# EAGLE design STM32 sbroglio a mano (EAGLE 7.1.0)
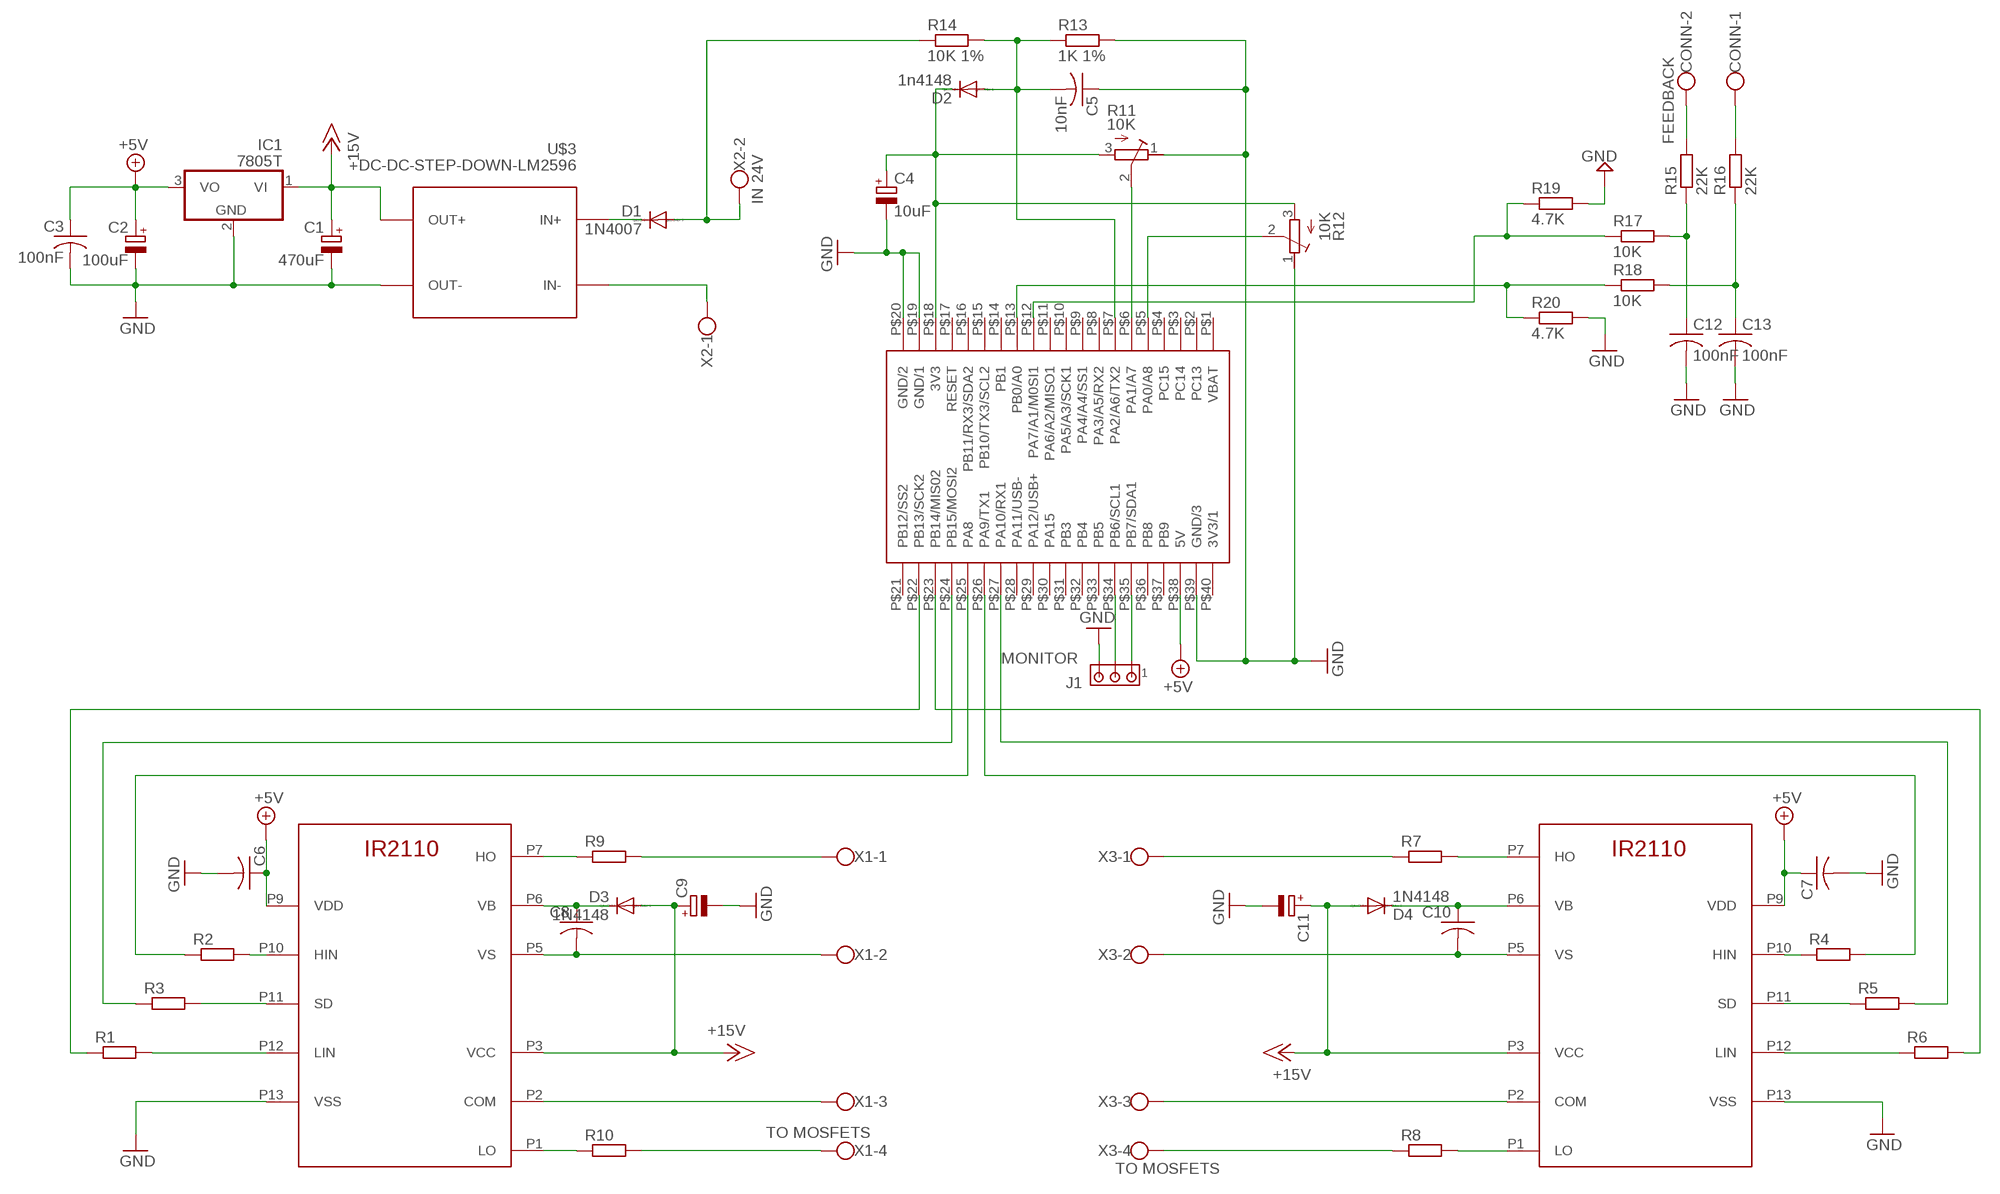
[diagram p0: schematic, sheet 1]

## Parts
C1  470uF  CPOL-EUE5-10.5  [E5-10,5]
C2  100uF  CPOL-EUE5-10.5  [E5-10,5]
C3  100nF  C-US050-025X075  [C050-025X075]
C4  10uF  CPOL-EUE3.5-8  [E3,5-8]
C5  10nF  C-US050-025X075  [C050-025X075]
C6  C-US050-025X075  [C050-025X075]
C7  C-US050-025X075  [C050-025X075]
C8  C-US050-025X075  [C050-025X075]
C9  CPOL-EUE3.5-8  [E3,5-8]
C10  C-US050-025X075  [C050-025X075]
C11  CPOL-EUE3.5-8  [E3,5-8]
C12  100nF  C-US050-025X075  [C050-025X075]
C13  100nF  C-US050-025X075  [C050-025X075]
CONN  FEEDBACK  W237-102  [W237-102]
D1  1N4007  1N4004  [DO41-10]
D2  1n4148  1N4004  [DO41-10]
D3  1N4148  1N4004  [DO41-10]
D4  1N4148  1N4004  [DO41-10]
IC1  7805T  [TO220H]
J1  MONITOR  MTA03-100  [10X03MTA]
R1  R-EU_0204/5  [0204/5]
R2  R-EU_0204/5  [0204/5]
R3  R-EU_0204/5  [0204/5]
R4  R-EU_0204/5  [0204/5]
R5  R-EU_0204/5  [0204/5]
R6  R-EU_0204/5  [0204/5]
R7  R-EU_0204/5  [0204/5]
R8  R-EU_0204/5  [0204/5]
R9  R-EU_0204/5  [0204/5]
R10  R-EU_0204/5  [0204/5]
R11  10K  R-TRIMMT93YB  [RTRIMT93YB]
R12  10K  R-TRIMMT93YA  [RTRIMT93YA]
R13  1K 1%  R-EU_0204/5  [0204/5]
R14  10K 1%  R-EU_0204/5  [0204/5]
R15  22K  R-EU_0204/5  [0204/5]
R16  22K  R-EU_0204/5  [0204/5]
R17  10K  R-EU_0204/5  [0204/5]
R18  10K  R-EU_0204/5  [0204/5]
R19  4.7K  R-EU_0204/5  [0204/5]
R20  4.7K  R-EU_0204/5  [0204/5]
U$1  IR2110N  [DIL14-1]
U$2  IR2110N  [DIL14-1]
U$3  DC-DC-STEP-DOWN-LM2596  [DC-DC-STEP-DOWN-LM2596]
U$4  BLUEPILL  [40-DIP-BLUE-PIL]
X1  TO MOSFETS  W237-4  [W237-4]
X2  IN 24V  W237-102  [W237-102]
X3  TO MOSFETS  W237-4  [W237-4]

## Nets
+5V: C2.+ C3.1 C6.1 C7.1 IC1.3(VO) U$1.P9(VDD) U$2.P9(VDD) U$4.P$38(5V)
+15V: C1.+ C9.+ C11.+ D3.A D4.A IC1.1(VI) U$1.P3(VCC) U$2.P3(VCC) U$3.OUT+
GND: C1.- C2.- C3.2 C4.- C5.1 C6.2 C7.2 C9.- C11.- C12.2 C13.2 IC1.2(GND) J1.3 R11.1(E) R12.1(E) R13.2 R19.2 R20.2 U$1.P13(VSS) U$2.P13(VSS) U$3.OUT- U$4.P$19(GND/1) U$4.P$20(GND/2) U$4.P$39(GND/3)
N$1: R2.2 U$1.P10(HIN)
N$2: R3.2 U$1.P11(SD)
N$3: R1.2 U$1.P12(LIN)
N$4: R4.1 U$2.P10(HIN)
N$5: R5.1 U$2.P11(SD)
N$6: R6.1 U$2.P12(LIN)
N$7: R2.1 U$4.P$25(PA8)
N$8: R1.1 U$4.P$22(PB13/SCK2)
N$9: R3.1 U$4.P$24(PB15/MOSI2)
N$10: R4.2 U$4.P$26(PA9/TX1)
N$11: R6.2 U$4.P$23(PB14/MIS02)
N$12: R5.2 U$4.P$27(PA10/RX1)
N$13: D1.A R14.1 X2.2
N$14: R9.1 U$1.P7(HO)
N$15: R10.1 U$1.P1(LO)
N$16: R8.2 U$2.P1(LO)
N$17: R7.2 U$2.P7(HO)
N$18: R12.2(S) U$4.P$5(PA0/A8)
N$19: R11.2(S) U$4.P$6(PA1/A7)
N$20: D1.C U$3.IN+
N$21: U$3.IN- X2.1
N$22: C4.+ D2.C R11.3(A) R12.3(A) U$4.P$18(3V3)
N$23: C5.2 D2.A R13.1 R14.2 U$4.P$7(PA2/A6/TX2)
N$24: C8.1 D3.C U$1.P6(VB)
N$25: C8.2 U$1.P5(VS) X1.2
N$26: R9.2 X1.1
N$27: U$1.P2(COM) X1.3
N$28: R10.2 X1.4
N$29: C10.1 D4.C U$2.P6(VB)
N$30: C10.2 U$2.P5(VS) X3.2
N$31: R7.1 X3.1
N$33: R8.1 X3.4
N$34: C12.1 R15.1 R17.2
N$35: C13.1 R16.1 R18.2
N$36: R18.1 R20.1 U$4.P$13(PB0/A0)
N$37: R17.1 R19.1 U$4.P$12(PA7/A1/M0SI1)
N$38: J1.2 U$4.P$34(PB6/SCL1)
N$39: J1.1 U$4.P$35(PB7/SDA1)
N$40: U$2.P2(COM) X3.3
N$42: CONN.2 R15.2
N$43: CONN.1 R16.2
Unconnected: U$4.P$1(VBAT) U$4.P$2(PC13) U$4.P$3(PC14) U$4.P$4(PC15) U$4.P$8(PA3/A5/RX2) U$4.P$9(PA4/A4/SS1) U$4.P$10(PA5/A3/SCK1) U$4.P$11(PA6/A2/MISO1) U$4.P$14(PB1) U$4.P$15(PB10/TX3/SCL2) U$4.P$16(PB11/RX3/SDA2) U$4.P$17(RESET) U$4.P$21(PB12/SS2) U$4.P$28(PA11/USB-) U$4.P$29(PA12/USB+) U$4.P$30(PA15) U$4.P$31(PB3) U$4.P$32(PB4) U$4.P$33(PB5) U$4.P$36(PB8) U$4.P$37(PB9) U$4.P$40(3V3/1)

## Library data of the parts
C1 = rcl:CPOL-EU: POLARIZED CAPACITOR, European symbol
C2 C4 C9 C11 = resistor modified:CPOL-EU: POLARIZED CAPACITOR, European symbol
C3 C5-C8 C10 C12 C13 = resistor modified:C-US: CAPACITOR, American symbol
CONN X2 = con-wago-500 modified:W237-102: WAGO SCREW CLAMP; MPN: 237-102; OC_FARNELL: unknown; OC_NEWARK: 70K9898
D1-D4 = diodemodified:1N4004: DIODE
IC1 = linear:78*: Positive VOLTAGE REGULATOR Source: http://cache.national.com/ds/LM/LM78L05.pdf http://www.fairchildsemi.com/ds/LM/LM7805.pdf
J1 = con-amp:MTA03-100: AMP connector
R1-R10 R13-R20 = resistor0305:R-EU_: RESISTOR, European symbol
R11 R12 = resistor modified:R-TRIMM: Trimm resistor
U$1 U$2 = jfw-pwm1:IR2110
U$3 = diy-modules:DC-DC-STEP-DOWN-LM2596: DC/DC Step-Down Regulator based on LM2596-ADJ chip LM2596 datasheet available here: http://www.ti.com/lit/ds/symlink/lm2596.pdf Click here to find device on ebay.com
U$4 = maplemini:BLUEPILL
X1 X3 = con-wago-500 modified:W237-4: WAGO SCREW CLAMP; OC_FARNELL: unknown; OC_NEWARK: unknown

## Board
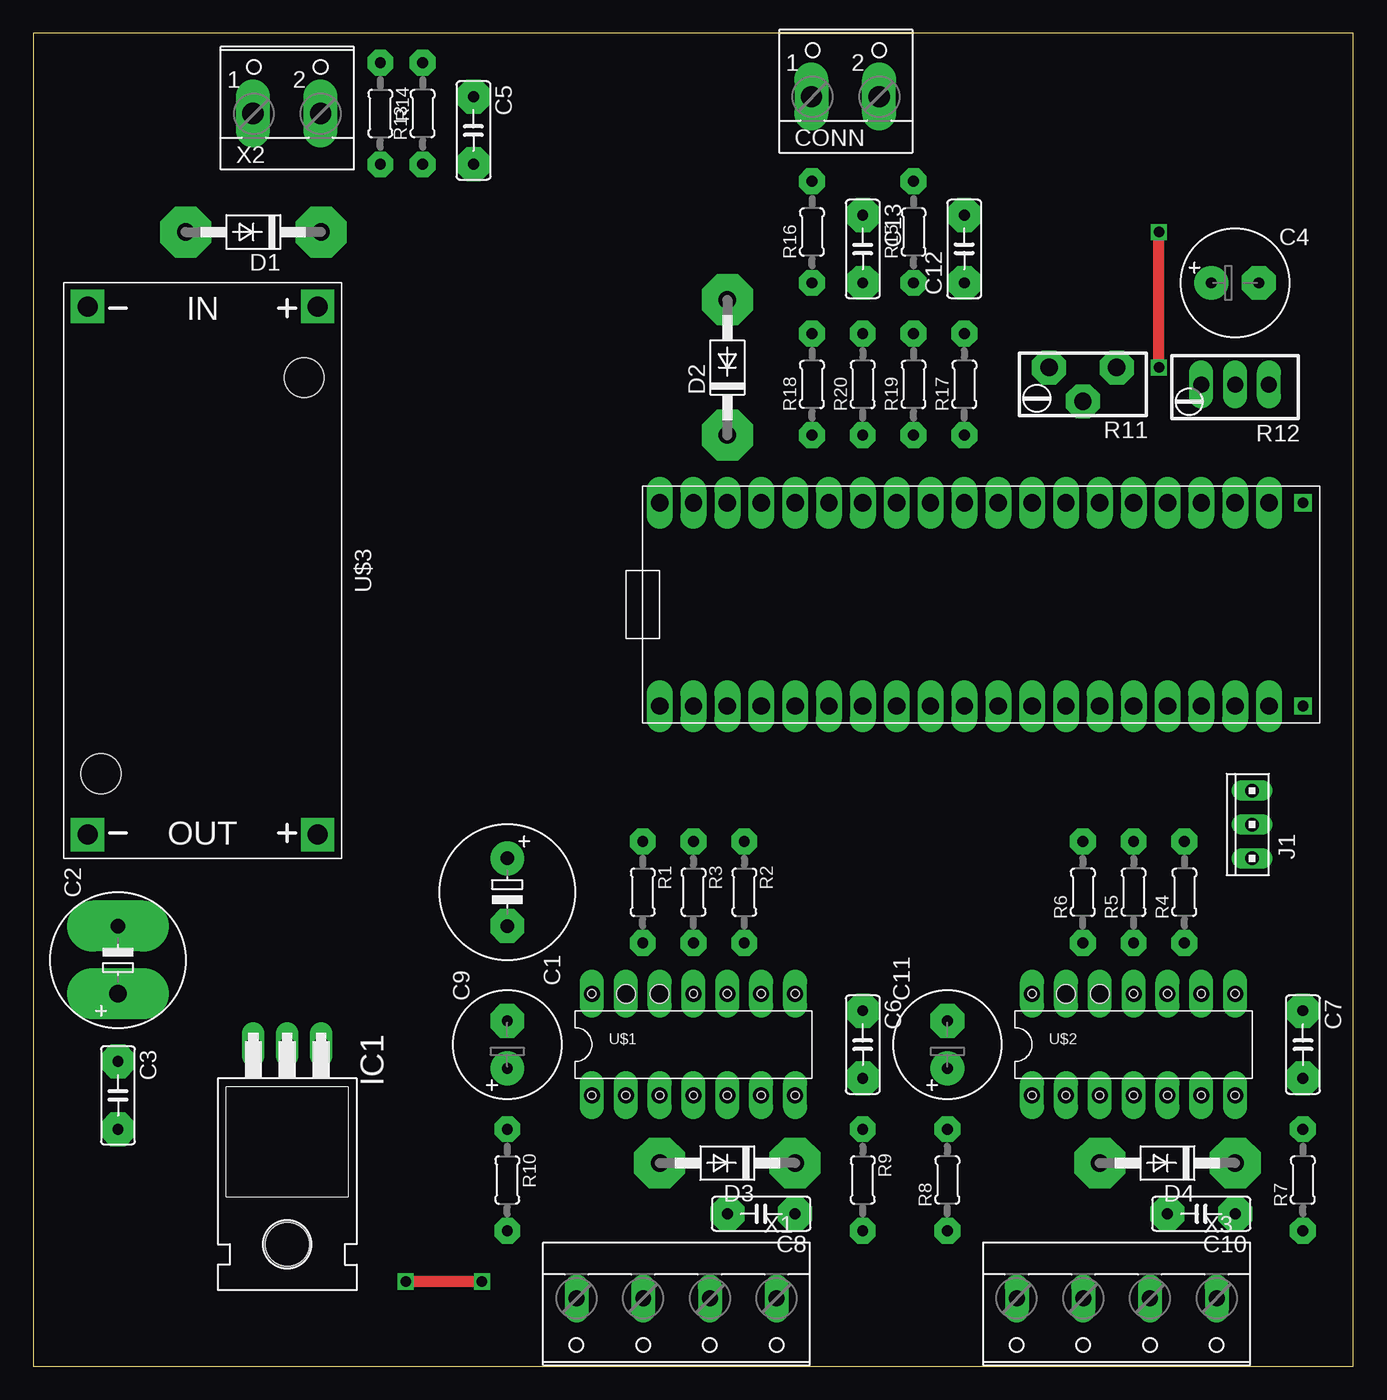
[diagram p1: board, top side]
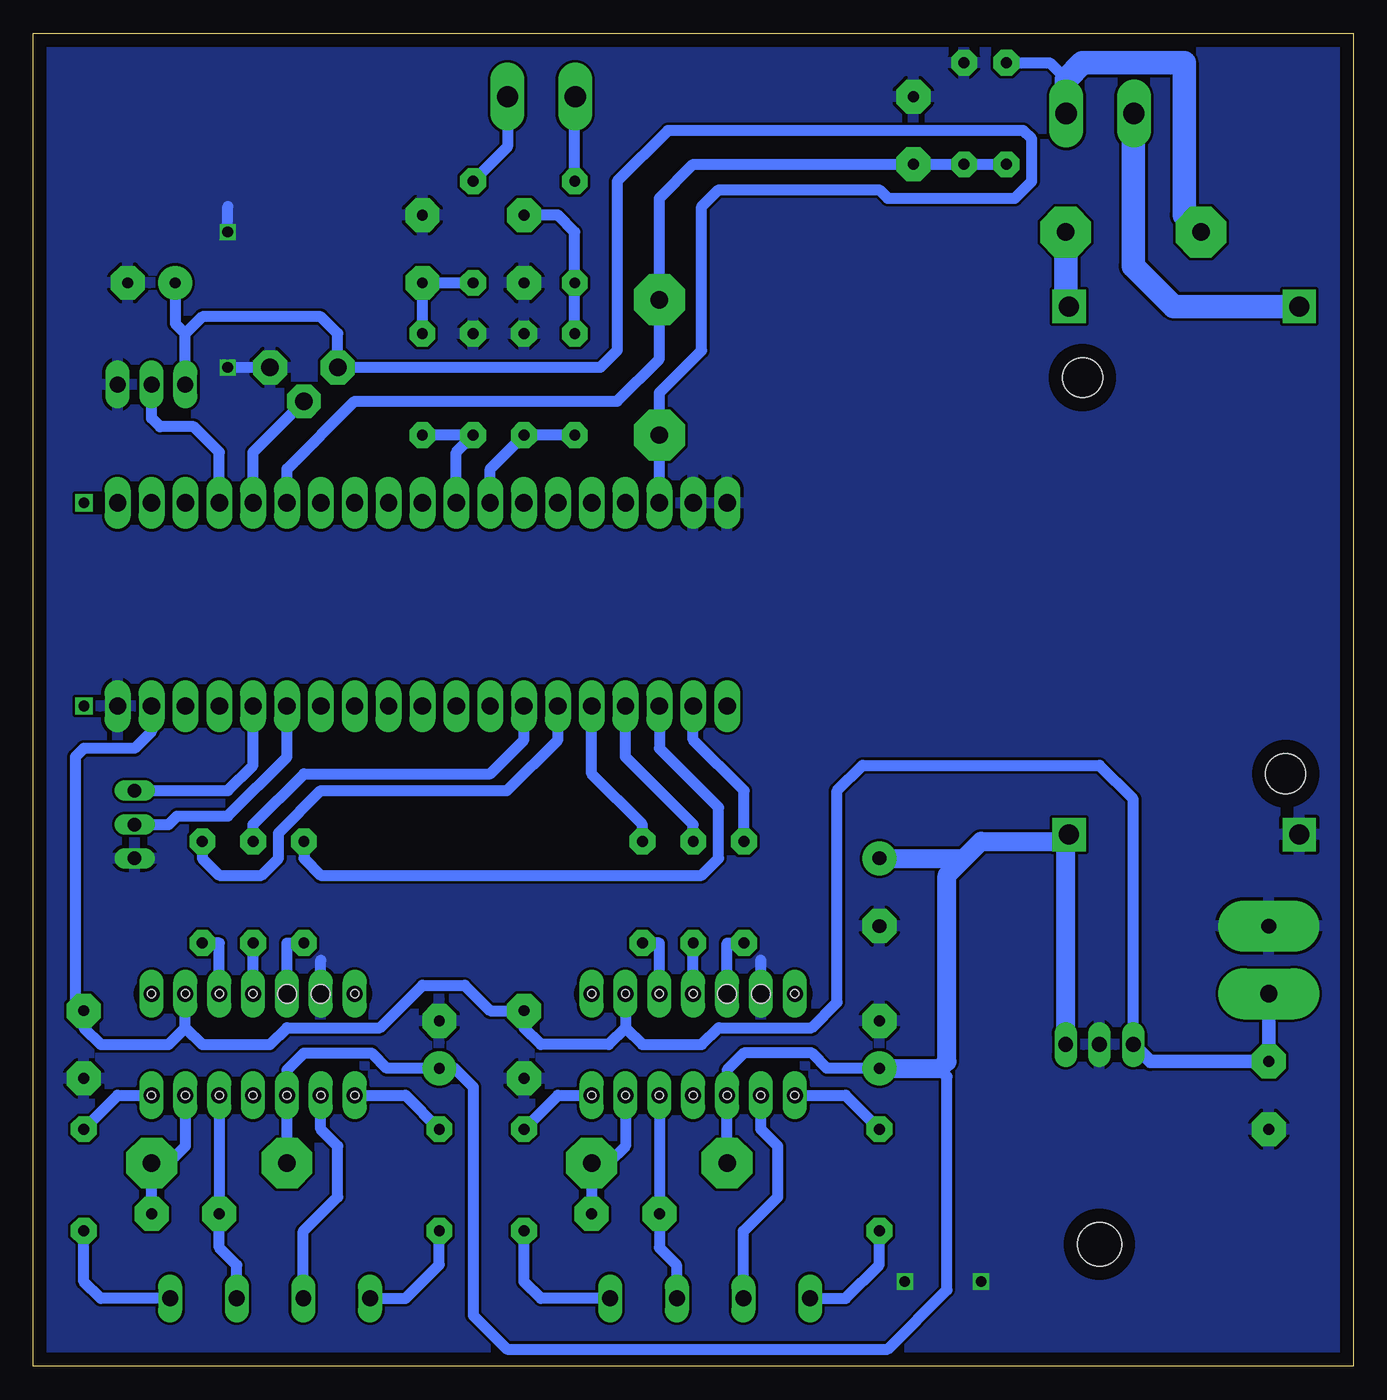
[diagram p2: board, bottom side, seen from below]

Size 99.04 x 100 mm. Coordinates in mm from the lower left corner, seen from the top.
Outline: 0,0 99.04,0 99.04,100 0,100 0,0
Copper layers (1*16): Top 0.035mm / dielectric 1.5mm / Bottom 0.035mm
Design rules "default": minimum track width 10mil, minimum drill 24mil, track to track 8mil, track to pad 8mil, pad to pad 8mil, via to via 8mil, smd to smd 8mil, copper to edge 40mil, drill to drill 8mil, minimum pad ring 10mil, minimum via ring 8mil, stop-mask expansion 4mil, vias tented up to drill 0mil, thermal gap 10mil

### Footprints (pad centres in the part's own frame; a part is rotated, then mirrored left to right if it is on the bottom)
E5-10,5 = drill 1.016 pad 2.54: + -2.54,0 | drill 1.016 pad 2.54 octagon: - 2.54,0
E5-10,5' = drill 1.3 pad 3.81 long: + -2.54,0 | drill 1.1 pad 3.81 long: - 2.54,0
C050-025X075 = drill 0.813 pad 2.54 octagon: 1 -2.54,0; 2 2.54,0
E3,5-8 = drill 0.813 pad 2.54: + -1.778,0 | drill 0.813 pad 2.54 octagon: - 1.778,0
W237-102 = drill 1.6 pad 2.54 long: 1 -2.58,-1.27; 2 2.5,-1.27
DO41-10 = drill 1.3 pad 3.81 octagon: A 5.08,0; C -5.08,0
TO220H = drill 1.118 long: 1 -2.54,-10.16; 2 0,-10.16; 3 2.54,-10.16 | hole 3.302: 0,4.826
10X03MTA = drill 1.016 long: 1 2.54,0; 2 0,0; 3 -2.54,0
0204/5 = drill 0.813 pad 1.93 octagon: 1 -3.81,0; 2 3.81,0
RTRIMT93YB = drill 1.3 pad 2.54 octagon: 1 1.27,-2.54; 2 -1.27,0; 3 1.27,2.54
RTRIMT93YA = drill 1.2 pad 1.778 long: 1 0,-2.54; 2 0,0; 3 0,2.54
DIL14-1 = drill 1.2 pad 1.778 long: P1 -8.89,-3.81; P2 -6.35,-3.81; P3 -3.81,-3.81; P4 -1.27,-3.81; P5 1.27,-3.81; P6 3.81,-3.81; P7 6.35,-3.81; P8 6.35,3.81; P9 3.81,3.81; P10 1.27,3.81; P11 -1.27,3.81; P12 -3.81,3.81; P13 -6.35,3.81; P14 -8.89,3.81 | hole 0.61: -8.89,-3.81; -6.35,-3.81; -3.81,-3.81; -1.27,-3.81; 1.27,-3.81; 3.81,-3.81; 6.35,-3.81; 6.35,3.81; 3.81,3.81; 1.27,3.81; -1.27,3.81; -8.89,3.81 | hole 1.4: -3.81,3.81; -6.35,3.81
DC-DC-STEP-DOWN-LM2596 = drill 1.5 pad 2.5 square: IN+ -19.812,8.636; IN- -19.812,-8.636; OUT+ 19.812,8.636; OUT- 19.812,-8.636 | hole 3: -14.478,7.62; 15.24,-7.62
40-DIP-BLUE-PIL = drill 0.8 square: P$1 -7.62,22.86; P$40 7.62,22.86 | drill 1.3 pad 1.676 long: P$2 -7.62,20.32; P$3 -7.62,17.78; P$4 -7.62,15.24; P$5 -7.62,12.7; P$6 -7.62,10.16; P$7 -7.62,7.62; P$8 -7.62,5.08; P$9 -7.62,2.54; P$10 -7.62,0; P$11 -7.62,-2.54; P$12 -7.62,-5.08; P$13 -7.62,-7.62; P$14 -7.62,-10.16; P$15 -7.62,-12.7; P$16 -7.62,-15.24; P$17 -7.62,-17.78; P$18 -7.62,-20.32; P$19 -7.62,-22.86; P$20 -7.62,-25.4; P$21 7.62,-25.4; P$22 7.62,-22.86; P$23 7.62,-20.32; P$24 7.62,-17.78; P$25 7.62,-15.24; P$26 7.62,-12.7; P$27 7.62,-10.16; P$28 7.62,-7.62; P$29 7.62,-5.08; P$30 7.62,-2.54; P$31 7.62,0; P$32 7.62,2.54; P$33 7.62,5.08; P$34 7.62,7.62; P$35 7.62,10.16; P$36 7.62,12.7; P$37 7.62,15.24; P$38 7.62,17.78; P$39 7.62,20.32
W237-4 = drill 1.194 long: 1 -7.5,-1.27; 2 -2.5,-1.27; 3 2.5,-1.27; 4 7.5,-1.27

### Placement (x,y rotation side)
C1  35.56,35.56 270 top
C2  100uF  [E5-10,5']  6.35,30.48 90 top
C3  6.35,20.32 270 top
C4  90.17,81.28 0 top
C5  33.02,92.71 270 top
C6  62.23,24.13 270 top
C7  95.25,24.13 270 top
C8  54.61,11.43 180 top
C9  35.56,24.13 90 top
C10  87.63,11.43 180 top
C11  68.58,24.13 90 top
C12  69.85,83.82 90 top
C13  62.23,83.82 270 top
CONN  60.96,96.52 0 top
D1  16.51,85.09 180 top
D2  52.07,74.93 90 top
D3  52.07,15.24 180 top
D4  85.09,15.24 180 top
IC1  19.05,13.97 180 top
J1  91.44,40.64 90 top
R1  45.72,35.56 270 top
R2  53.34,35.56 270 top
R3  49.53,35.56 270 top
R4  86.36,35.56 90 top
R5  82.55,35.56 90 top
R6  78.74,35.56 90 top
R7  95.25,13.97 90 top
R8  68.58,13.97 90 top
R9  62.23,13.97 270 top
R10  35.56,13.97 270 top
R11  78.74,73.66 90 top
R12  90.17,73.66 90 top
R13  29.21,93.98 90 top
R14  26.04,93.98 270 top
R15  66.04,85.09 90 top
R16  58.42,85.09 90 top
R17  69.85,73.66 90 top
R18  58.42,73.66 90 top
R19  66.04,73.66 90 top
R20  62.23,73.66 90 top
U$1  50.8,24.13 0 top
U$2  83.82,24.13 0 top
U$3  12.7,59.69 270 top
U$4  72.39,57.15 270 top
X1  48.26,3.81 180 top
X2  19.05,95.25 0 top
X3  81.28,3.81 180 top

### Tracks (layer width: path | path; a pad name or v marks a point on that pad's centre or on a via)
+5V
  Bottom 0.813: 87.63,25.4 88.9,24.13 93.98,24.13 95.25,25.4 C7.1 95.89,27.3 95.89,45.72 95.25,46.35 91.44,46.35 90.17,47.62 U$4.P$38 | 87.63,25.4 U$2.P9 | U$1.P9 54.61,25.4 | 54.61,25.4 55.88,24.13 60.96,24.13 62.23,25.4 C6.1 64.77,26.67 66.67,28.57 69.85,28.57 73.03,25.4 80.01,25.4 81.28,24.13 86.36,24.13 87.63,25.4 | 54.61,25.4 53.34,24.13 48.9,24.13 47.62,25.4 40.64,25.4 38.73,27.3 38.73,43.18 36.83,45.09 19.05,45.09 16.51,42.55 IC1.3
  Bottom 1.016: C2.+ C3.1 15.24,22.86 IC1.3
+15V
  Bottom 0.813: D4.A U$2.P3 80.01,22.23 78.74,23.5 73.66,23.5 72.52,22.35 C11.+ 67.44,22.35 66.04,20.95 66.04,3.81 63.5,1.27 34.92,1.27 30.48,5.71 30.48,21.72 31.11,22.35 | D3.A U$1.P3 46.99,22.23 45.72,23.5 40.64,23.5 39.5,22.35 C9.+
  Bottom 1.422: IC1.1 21.59,39.62 | 21.59,39.62 U$3.OUT+ | C1.+ 29.21,38.1 | 29.21,38.1 27.94,39.37 21.84,39.37 21.59,39.62 | C9.+ 31.11,22.35 30.99,22.35 30.48,22.86 30.48,36.83 29.21,38.1
GND  (via drill 0.8)
  Top 0.813: v84.45,74.93 v84.45,85.09 | v33.66,6.35 v27.94,6.35
  Bottom 0.813: U$1.P13 44.45,30.48 | U$2.P13 77.47,30.48 | R11.1 v84.45,74.93 | v84.45,85.09 84.45,87
  pour Bottom: 0,0 0,100.33 99.06,100.33 99.06,0
N$1
  Bottom 0.813: U$1.P10 52.07,31.75 R2.2
N$2
  Bottom 0.813: U$1.P11 R3.2
N$3
  Bottom 0.813: U$1.P12 46.99,29.21 46.99,31.75 R1.2
N$4
  Bottom 0.813: U$2.P10 85.09,31.75 R4.1
N$5
  Bottom 0.813: U$2.P11 R5.1
N$6
  Bottom 0.813: U$2.P12 80.01,30.48 80.01,31.75 R6.1
N$7
  Bottom 0.813: R2.1 53.34,40.64 57.15,44.45 U$4.P$25
N$8
  Bottom 0.813: R1.1 45.72,43.18 49.53,46.99 U$4.P$22
N$9
  Bottom 0.813: R3.1 49.53,40.64 54.61,45.72 U$4.P$24
N$10
  Bottom 0.813: R4.2 86.36,38.1 85.09,36.83 81.92,36.83 80.64,38.1 80.64,40.01 77.47,43.18 63.5,43.18 59.69,46.99 U$4.P$26
N$11
  Bottom 0.813: U$4.P$23 52.07,46.35 47.62,41.91 47.62,38.1 48.9,36.83 77.47,36.83 78.74,38.1 R6.2
N$12
  Bottom 0.813: R5.2 82.55,40.64 78.74,44.45 64.77,44.45 62.23,46.99 U$4.P$27
N$13
  Bottom 0.813: R14.1 22.78,97.79 21.55,96.56
  Bottom 1.778: X2.2 21.55,96.56 20.32,97.79 12.7,97.79 12.7,86.36 D1.A
N$14
  Bottom 0.813: R9.1 59.69,20.32 U$1.P7
N$15
  Bottom 0.813: U$1.P1 38.1,20.32 R10.1
N$16
  Bottom 0.813: U$2.P1 71.12,20.32 R8.2
N$17
  Bottom 0.813: R7.2 92.71,20.32 U$2.P7
N$18
  Bottom 0.813: U$4.P$5 85.09,68.58 87,70.48 89.53,70.48 90.17,71.12 R12.2
N$19
  Bottom 0.813: U$4.P$6 82.55,68.58 R11.2
N$20
  Bottom 1.778: D1.C 21.59,79.76 U$3.IN+
N$21
  Bottom 1.778: X2.1 16.51,93.98 16.51,82.55 13.46,79.5 U$3.IN-
N$22
  Bottom 0.813: U$4.P$18 D2.C 52.07,73.03 48.9,76.2 48.9,87 47.62,88.27 35.56,88.27 34.92,87.63 25.4,87.63 24.13,88.9 24.13,92.08 24.77,92.71 51.44,92.71 55.24,88.9 55.24,76.2 56.52,74.93 R11.3 76.2,77.47 77.47,78.74 86.36,78.74 87.63,77.47 | R12.3 87.63,77.47 | C4.+ 88.39,78.23 87.63,77.47
N$23
  Bottom 0.813: R14.2 R13.1 C5.2 49.53,90.17 52.07,87.63 D2.A 52.07,75.56 55.24,72.39 74.93,72.39 80.01,67.31 U$4.P$7
N$24
  Bottom 0.813: U$1.P6 54.61,16.51 55.88,15.24 D3.C C8.1
N$25
  Bottom 0.813: U$1.P5 C8.2 52.07,8.89 50.8,7.62 50.8,5.12 X1.2
N$26
  Bottom 0.813: X1.1 60.96,5.08 62.23,6.35 R9.2
N$27
  Bottom 0.813: X1.3 45.76,10.12 43.18,12.7 43.18,16.51 44.45,17.78 U$1.P2
N$28
  Bottom 0.813: X1.4 38.1,5.08 35.56,7.62 R10.2
N$29
  Bottom 0.813: U$2.P6 87.63,16.51 88.9,15.24 D4.C C10.1
N$30
  Bottom 0.813: U$2.P5 C10.2 85.09,8.89 83.78,7.58 X3.2
N$31
  Bottom 0.813: X3.1 93.98,5.08 95.25,6.35 R7.1
N$33
  Bottom 0.813: X3.4 71.12,5.08 68.58,7.62 R8.1
N$34
  Bottom 0.813: R17.2 C12.1 R15.1
N$35
  Bottom 0.813: R18.2 R16.1 58.42,85.09 59.69,86.36 C13.1
N$36
  Bottom 0.813: U$4.P$13 64.77,67.31 R20.1 R18.1
N$37
  Bottom 0.813: U$4.P$12 67.31,68.58 R19.1 R17.1
N$38
  Bottom 0.813: J1.2 88.9,40.64 88.27,41.27 84.45,41.27 80.01,45.72 U$4.P$34
N$39
  Bottom 0.813: J1.1 84.45,43.18 82.55,45.09 U$4.P$35
N$40
  Bottom 0.813: X3.3 78.78,10.12 76.2,12.7 76.2,16.51 77.47,17.78 U$2.P2
N$42
  Bottom 0.813: R15.2 63.46,91.48 CONN.2
N$43
  Bottom 0.813: R16.2 58.42,95.21 CONN.1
